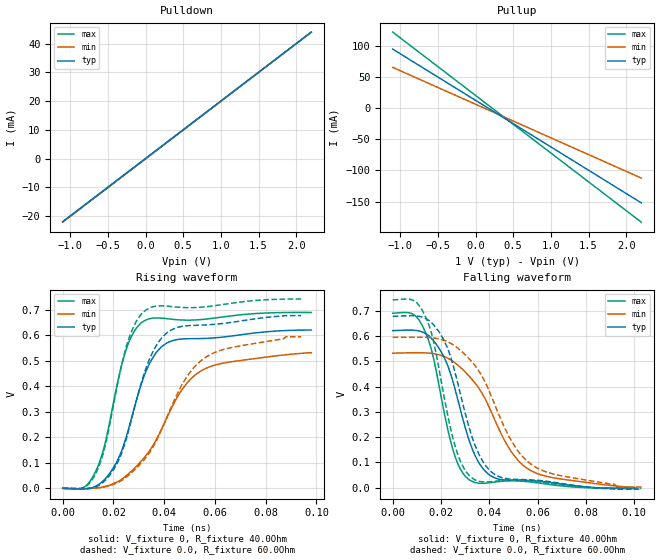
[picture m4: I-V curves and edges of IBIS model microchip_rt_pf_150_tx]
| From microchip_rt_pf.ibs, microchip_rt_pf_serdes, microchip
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|   MODEL microchip_rt_pf_150_tx
[Model] microchip_rt_pf_150_tx
Model_type   Output
Polarity   Non-Inverting
Enable   Active-High
Vmeas = 0.5
|   typ   min   max
C_comp   0.407p  0.407p  0.407p
[Voltage Range]   1.0  0.9  1.1
[Temperature Range]   60   100   0
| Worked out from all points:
|   slope of the pulldown table from 0 to 0.15 V, typ, clamps not added: 50.1 ohm
|   slope of the pullup table from 0 to 0.15 V, typ, clamps not added: 13.3 ohm
|   rising waveform, V_fixture 0, R_fixture 40.0Ohm: 20-80 % time 12.4ps typ, 19.2ps min, 9.61ps max; typ from 0 V to 0.621 V
|   rising waveform, V_fixture 0.0, R_fixture 60.0Ohm: 20-80 % time 12.8ps typ, 19.3ps min, 10ps max; typ from 0 V to 0.678 V
|   falling waveform, V_fixture 0, R_fixture 40.0Ohm: 20-80 % time 12.3ps typ, 18.9ps min, 9.52ps max; typ from 0.621 V to -0.004 V
|   falling waveform, V_fixture 0.0, R_fixture 60.0Ohm: 20-80 % time 12.6ps typ, 19.4ps min, 9.92ps max; typ from 0.678 V to -0.006 V
[Pullup]
|   X   TYP   MIN   MAX
-1.1V     95.29mA    65.91mA    122.6mA
1.01V     -62.89mA   -47.99mA   -72.9mA
1.089V    -68.78mA   -52.23mA   -80.18mA
2.2V      -152.1mA   -112.2mA   -183.2mA
[Pulldown]
|   X   TYP   MIN   MAX
-1.1V     -21.87mA   -22.06mA   -21.96mA
1.01V     20.25mA    20.18mA    20.22mA
1.021V    20.48mA    20.41mA    20.44mA
2.2V      44mA       44mA       44mA
[Ramp]
R_load = 50.0Ohm
|   typ   min   max
dV/dt_r   3.73E-1V/1.24E-2ns   3.19E-1V/1.92E-2ns   4.14E-1V/9.62E-3ns
dV/dt_f   3.75E-1V/1.23E-2ns   3.18E-1V/1.89E-2ns   4.15E-1V/9.52E-3ns
[Rising Waveform]
V_fixture   = 0
V_fixture_min = 0
V_fixture_max = 0
R_fixture   = 40.0Ohm
|   Time   V(typ)   V(min)   V(max)
0s        0V         0V         0V
8ps       -2.049mV   -1.289mV   2.472mV
13ps      8.05mV     932.7uV    66.58mV
17ps      39.69mV    7.858mV    188.5mV
22ps      118.2mV    27.72mV    432.1mV
26ps      234.4mV    57.74mV    572.2mV
31ps      409.7mV    107.2mV    650.2mV
39ps      556.2mV    232.8mV    667.9mV
54ps      587.7mV    457.6mV    662.1mV
98ps      621.5mV    532.3mV    690.3mV
[Rising Waveform]
V_fixture   = 0.0
V_fixture_min = 0.0
V_fixture_max = 0.0
R_fixture   = 60.0Ohm
|   Time   V(typ)   V(min)   V(max)
0s        0V         0V         0V
9ps       -2.295mV   -490uV     5.374mV
14ps      10.07mV    1.909mV    79.22mV
21ps      88.76mV    19.6mV     379mV
25ps      191.8mV    43.39mV    554.1mV
33ps      476.3mV    123.8mV    701.4mV
41ps      609.8mV    277.7mV    715.3mV
48ps      637.1mV    423.1mV    709.6mV
55ps      640.9mV    504.9mV    711.3mV
94ps      678mV      595.1mV    742.9mV
[Falling Waveform]
V_fixture   = 0
V_fixture_min = 0
V_fixture_max = 0
R_fixture   = 40.0Ohm
|   Time   V(typ)   V(min)   V(max)
0s        621.5mV    532.3mV    690.3mV
8ps       623.4mV    533.9mV    688.6mV
13ps      613.1mV    533.8mV    626.7mV
17ps      581.1mV    530mV      508.9mV
25ps      419mV      500mV      148.8mV
32ps      178mV      437.7mV    29.29mV
40ps      50.7mV     317.6mV    19.49mV
48ps      29.17mV    159.5mV    27.04mV
55ps      28.55mV    81.41mV    24.8mV
100ps     -3.933mV   1.663mV    -1.335mV
[Falling Waveform]
V_fixture   = 0.0
V_fixture_min = 0.0
V_fixture_max = 0.0
R_fixture   = 60.0Ohm
|   Time   V(typ)   V(min)   V(max)
0s        678mV      595.1mV    742.9mV
9ps       680.2mV    595.1mV    738.8mV
14ps      667.6mV    594.6mV    667.2mV
23ps      546.1mV    576.2mV    276.7mV
27ps      411.6mV    551.5mV    130.1mV
32ps      227.3mV    506.7mV    45.32mV
41ps      61.47mV    358.7mV    24.03mV
48ps      34.86mV    205mV      30.61mV
57ps      31.19mV    95.34mV    27.44mV
103ps     -5.738mV   2.66mV     -1.419mV
[Algorithmic Model]
Executable Linux_gcc5.4_64   MPF300T-TX_LX64.so   MPF300T-TX-R150.ami
Executable Windows_cl18.00.40629_64 MPF300T-TX_WIN64.dll  MPF300T-TX-R150.ami
Executable Windows_cl18.00.40629_32 MPF300T-TX_WIN32.dll  MPF300T-TX-R150.ami
[End Algorithmic Model]
